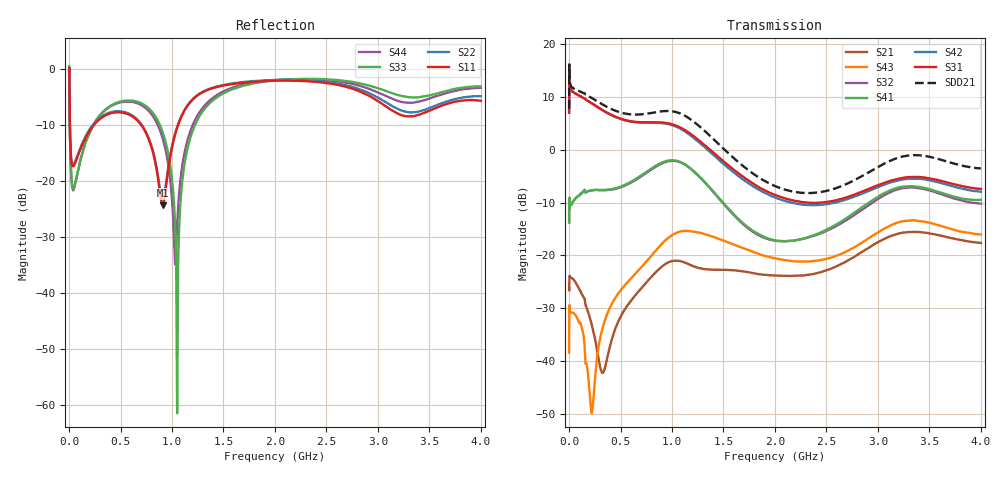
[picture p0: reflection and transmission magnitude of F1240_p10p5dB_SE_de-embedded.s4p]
! Integrated Device Technology
! Corporate Headquarters
! 6024 Silver Creek Valley Road
! San Jose, CA 95138  USA
! Phone:  1-408-284-8200
! Toll Free:  1-800-223-1366
! Webpage:  http://www.idt.com/
! Timing and RF Division
! 515 Groton Road, Suite 102
! Westford, MA 01886-6024
! Device:  F1240
! Description: Dual Intermediate Frequency Digital Variable Gain Amplifier
! Frequency:  10.0 -  500.00 MHz
! Package:  5x5 mm QFN Plastic Package: 32 pin
! Ports:  8 RF, 20 DC
!  Pin  1  = GA3 / Data  Pin 17  = RF OUT_B+
!  Pin  2  = GA4 / CLK  Pin 18  = RF OUT_B-
!  Pin  3  = GA5  Pin 19  = STBY_B
!  Pin  4  = VMODE  Pin 20  = Ground
!  Pin  5  = No Connect  Pin 21  = Ground
!  Pin  6  = GB5  Pin 22  = STB_A
!  Pin  7  = GB4  Pin 23  = RF OUT_A-  = Port 4
!  Pin  8  = GB3  Pin 24  = RF OUT_A+  = Port 3
!  Pin  9  = GB2  Pin 25  = GA0
!  Pin 10  = GB1  Pin 26  = ISET_A
!  Pin 11  = RF IN_B+  Pin 27  = VCC
!  Pin 12  = RF IN_B-  Pin 28  = Ground
!  Pin 13  = Ground  Pin 29  = RF IN_A-  = Port 2
!  Pin 14  = VCC  Pin 30  = RF IN_A+  = Port 1
!  Pin 15  = ISET_B  Pin 31  = GA1
!  Pin 16  = GB0  Pin 32  = GA2 / CSb
! Gain  = +19.5 dB
! State  = 1
! Voltage  = +5.00 V
! Current  = 85.292 mA (one channel only)
! Temperture  =  +25 C
! Test Date  =  2017-10-18
! Board  =  EB4031
! Data:  The device was measured on a custom evaluation board which has
!  individual transmission lines to the RF pins.  Data was collected
!  using a calibrated network analyzer.  The evaluation board was
!  de-embedded using Automatic Fixture Removal.
!  The reference plane is the edge of the package pin.
!  Only Channel A was measured.
!  This data is in single-ended operation.  If your needs are balanced
!  or differential S-parameters then this file needs to be used a
!  linear simulator.
! File Date:  2017-11-10  MJV
! Note:
!  Integrated Device Technology supplies this data as a sample of measured
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# Hz S dB R 100
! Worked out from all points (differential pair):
!   410 points, 500 kHz to 4 GHz, reference 100 ohm
!   strongest paths, dB at 500 kHz, 930 MHz, 1.96 GHz, 2.98 GHz, 4 GHz:
!     S31: 7.0, 5.1, -8.2, -6.9, -7.4
!     S42: 7.0, 5.0, -8.7, -7.3, -7.9
!     S41: -13.8, -2.2, -17.0, -9.2, -9.5
!     S32: -13.7, -2.4, -17.1, -9.6, -10.2
!     S43: -38.4, -17.3, -20.4, -15.9, -16.0
!     S21: -26.2, -21.7, -23.8, -17.7, -17.7
!   taken as a pair (ports 1,2 in; 3,4 out), SDD21 dB: 7.8, 7.3, -6.5, -3.5, -3.5
!   lowest |S11| = -24.4 dB at 910 MHz (marker M1), VSWR 1.13, Z = 111 + j6.82 ohm
!   |S11| at or under -10 dB: 7.79 MHz to 243.2 MHz (235.4 MHz wide, 188 % of centre); 699.2 MHz to 1.059 GHz (360.2 MHz wide, 41 % of centre)
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500000  -0.38 -5.7  -26.21 -3.2  -27.21 81.1  -58.63 68.4
        -26.19 -3.1  -0.38 -5.7  -58.77 69.6  -27.21 82.3
        7.01 -105.1  -13.72 67.7  -0.47 1.4  -38.44 -119.4
        -13.81 68.8  6.99 -104.0  -38.40 -118.7  -0.48 3.7
3000000  -3.10 -60.6  -25.11 3.7  -16.44 22.4  -45.98 66.3
         -25.10 3.7  -3.06 -60.5  -45.91 65.5  -16.45 22.5
         14.99 -178.9  -9.68 -7.5  -2.60 -56.3  -29.45 71.1
         -9.60 -7.5  14.99 -178.7  -29.42 71.2  -2.66 -56.0
2e8  -11.07 -133.5  -31.56 -76.9  -18.60 -50.2  -34.43 12.8
     -31.67 -74.7  -10.80 -134.5  -34.39 13.4  -18.62 -50.3
     9.05 109.8  -7.78 -34.3  -11.36 -96.2  -42.72 -122.7
     -7.75 -34.7  9.02 109.1  -46.03 -119.7  -11.40 -95.1
5.3e8  -7.87 179.4  -31.34 -13.7  -19.80 -108.1  -28.58 -57.0
       -30.61 -16.2  -7.70 178.1  -28.70 -55.1  -19.92 -108.3
       5.69 26.5  -6.91 -98.4  -5.74 -157.1  -27.16 13.5
       -6.76 -99.9  5.63 25.6  -25.92 9.7  -5.91 -157.0
9.1e8  -24.36 30.5  -22.03 -83.5  -17.65 170.4  -25.03 -146.6
       -21.99 -91.3  -23.29 30.9  -25.28 -140.5  -17.96 169.8
       5.14 -68.5  -2.54 167.3  -11.35 138.0  -18.68 -67.3
       -2.37 163.2  5.01 -70.2  -17.64 -73.2  -12.48 140.0
1.52e9  -2.93 -150.4  -22.17 137.7  -23.80 28.3  -26.52 75.6
        -22.74 140.2  -2.83 -150.1  -26.29 81.2  -24.75 28.2
        -2.54 127.9  -10.70 -14.1  -4.20 -138.4  -17.79 127.3
        -10.55 -19.7  -3.03 126.8  -17.35 124.4  -3.87 -141.3
4e9  -5.73 -152.3  -17.74 75.6  -20.73 -60.6  -20.77 -48.0
     -17.65 75.0  -4.92 -148.7  -22.33 -28.6  -22.95 -52.9
     -7.42 17.0  -10.19 -102.5  -3.17 -138.8  -16.47 86.0
     -9.49 -115.7  -7.94 25.4  -16.04 60.6  -3.40 -145.5
